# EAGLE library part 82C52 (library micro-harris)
MICROCONTROLLER/MEMORY DEVICE
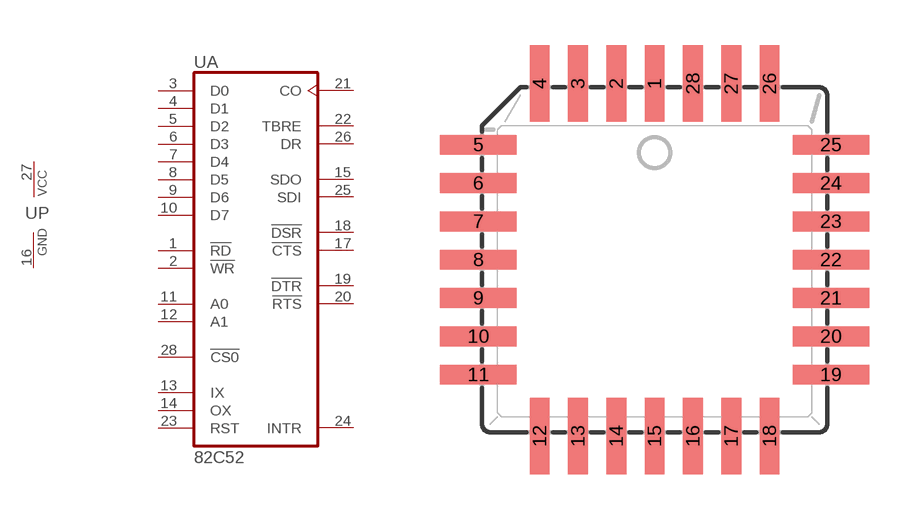
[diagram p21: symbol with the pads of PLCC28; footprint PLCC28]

Designator prefix U; gates A=82C52 P=PWRN

## 82C52 (MF: INTERSIL; MPN: IS82C52; OC_FARNELL: unknown; OC_NEWARK: 05B7416)  [PLCC28]
1  A:!RD  in
2  A:!WR  in
3  A:D0
4  A:D1
5  A:D2
6  A:D3
7  A:D4
8  A:D5
9  A:D6
10  A:D7
11  A:A0  in
12  A:A1  in
13  A:IX
14  A:OX
15  A:SDO  out
16  P:GND  pwr
17  A:!CTS  in
18  A:!DSR  in
19  A:!DTR  out
20  A:!RTS  out
21  A:CO  out
22  A:TBRE  out
23  A:RST  in
24  A:INTR  out
25  A:SDI  in
26  A:DR  out
27  P:VCC  pwr
28  A:!CS0  in

## Footprint PLCC28 (pad centres in mm)
PLASTIC LEADED CHIP CARRIER square
smd 0.66 x 2.54: 1 0,5.842; 2 -1.27,5.842; 3 -2.54,5.842; 4 -3.81,5.842; 12 -3.81,-5.842; 13 -2.54,-5.842; 14 -1.27,-5.842; 15 0,-5.842; 16 1.27,-5.842; 17 2.54,-5.842; 18 3.81,-5.842; 26 3.81,5.842; 27 2.54,5.842; 28 1.27,5.842
smd 2.54 x 0.66: 5 -5.842,3.81; 6 -5.842,2.54; 7 -5.842,1.27; 8 -5.842,0; 9 -5.842,-1.27; 10 -5.842,-2.54; 11 -5.842,-3.81; 19 5.842,-3.81; 20 5.842,-2.54; 21 5.842,-1.27; 22 5.842,0; 23 5.842,1.27; 24 5.842,2.54; 25 5.842,3.81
